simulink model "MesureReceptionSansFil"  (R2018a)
settings: Solver=FixedStepDiscrete  StartTime=0.0  StopTime=inf  FixedStep=0.01  RelTol=1e-3  EnableMultiTasking=on
undefined symbols (not defined in the file): a033, bd0f03049666, bf82, bf9c, f, f7e3, lineargauge, ReceptionUDP, sdiscope
libraries: instrumentlib x1

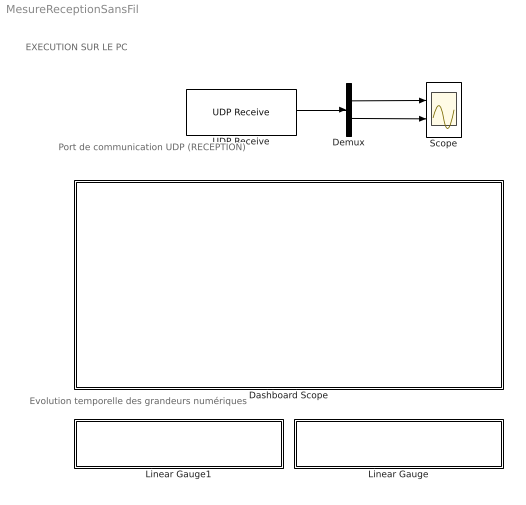
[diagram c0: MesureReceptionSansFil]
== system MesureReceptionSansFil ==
  note: Port de communication UDP (RECEPTION)
  note: Evolution temporelle des grandeurs numériques
  note: EXECUTION SUR LE PC
  Dashboard Scope : Subsystem  DialogController=hmiCreateDDGDialog  IsWebBlock=on  mask(MWDashboardBlock){webBlockId=8566b974-09f6-4800-a033-bd0f03049666, webBlockType=sdiscope, ShowInitialText=on, HMISrcModelName=ReceptionUDP}
      mask prompts: webBlockId "WebBlock Id"; webBlockType "WebBlock Type"; HMISrcModelName "Source Model"
      mask help: SimulinkHMI:dialogs:HMIScopeDialogDesc
  Demux : Demux  Outputs=2
  Linear Gauge : Subsystem  DialogController=hmiCreateDDGDialog  IsWebBlock=on  mask(MWDashboardBlock){webBlockId=18a26100-999b-40c7-bf82-65dc0b9ada4c, webBlockType=lineargauge, ShowInLibBrowser=on, ShowInitialText=on, HMISrcModelName=ReceptionUDP}
      mask prompts: webBlockId "WebBlock Id"; webBlockType "WebBlock Type"; HMISrcModelName "Source Model"
      mask help: SimulinkHMI:dialogs:LinearGaugeDialogDesc
  Linear Gauge1 : Subsystem  DialogController=hmiCreateDDGDialog  IsWebBlock=on  mask(MWDashboardBlock){webBlockId=45f58cdd-f7e3-4f04-bf9c-00a28107f757, webBlockType=lineargauge, ShowInLibBrowser=on, ShowInitialText=on, HMISrcModelName=ReceptionUDP}
      mask prompts: webBlockId "WebBlock Id"; webBlockType "WebBlock Type"; HMISrcModelName "Source Model"
      mask help: SimulinkHMI:dialogs:LinearGaugeDialogDesc
  Scope : Scope  NumInputPorts=2
  UDP Receive : instrumentlib/UDP Receive  Host=192.168.1.20  Port=50001  LocalPort=50002  EnablePortSharing=off  GetLatestData=off  DataSize=2  DataType=uint16  ASCIIFormatting=%f,  Terminator=LF  ByteOrder=LittleEndian  EnableBlockingMode=on  Timeout=10  SampleTime=0.01  LocalAddress=0.0.0.0
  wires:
  Demux/1 -> Scope/1
  Demux/2 -> Scope/2
  UDP Receive/1 -> Demux/1

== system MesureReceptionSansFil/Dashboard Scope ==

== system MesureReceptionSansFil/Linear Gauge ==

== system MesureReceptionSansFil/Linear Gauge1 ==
